| TEXAS INSTRUMENTS INCORPORATED
| Standard Linear and Logic Group
| IBIS Model of SN74CBT3125C
| QUADRUPLE FET BUS SWITCH WITH-2V UNDERSHOOT PROTECTION
| This file contains package information for the following:
|  SOIC 14-pin (D) package as [Component] CBT3125C_D
|  SSOP 14-pin (DB) package as [Component] CBT3125C_DB
|  TSSOP 14-pin (PW) package as [Component] CBT3125C_PW
|  SSOP 16-pin (DBQ) package as [Component] CBT3125C_DBQ
|  QFN 14-pin (RGY) package as [Component] CBT3125C_RGY
|  TVSOP 14-pin (DGV) package as [Component] CBT3125C_DGV
| This device can be powered at the following Vccs:
|  5 volt Vcc
|  4 volt Vcc
| This file provides unique models under the [Model Selector] for each Vcc.
| For operation at a specific Vcc, select the appropriate model after each
| [Model Selector] keyword.
[IBIS Ver]   3.2
[Comment char]  |_char
[File Name]   sn74cbt3125c.ibs
[File Rev]   1.1 | b_die
[Date]   JULY 9, 2003
[Source]   Data created from TI-SPICE simulations at TI-SLL.
[Notes]   The following is an IBIS list for the CBT3125C.
   Please contact sllibis@ti.com with questions and
   comments concerning SLL IBIS models.
   - The SSOP 16-pin package Component is commented out as
   there is different Series Pin Mapping.
   - Power-clamp data has been deleted since there is no
   power-clamp diode in the device.
   - Non-monotonic data due to FET characteristics.
[Disclaimer] Property of Texas Instruments Incorporated.  Unauthorized
   reproduction and/or distribution is strictly prohibited.
   This product is protected under copyright law.
   Created  2003, (C) Copyright  2003, Texas Instruments
   Incorporated, All Rights Reserved
   UNLESS THERE IS A SIGNED, WRITTEN AGREEMENT TO THE
   CONTRARY, TEXAS INSTRUMENTS (TI) IS PROVIDING THE IBIS
   MODELS  AND WITHOUT ANY WARRANTY, EXPRESSED OR
   IMPLIED.  TI assumes no liability for:
   1) the accuracy of the IBIS models provided to your
   company;
   2) the proper functioning of these IBIS Models in your
   design or for any resulting applications; or
   3) infringement of patents, copyrights or intellectual
   property rights resulting from your use of these IBIS
   models.
   TI provides IBIS Models as a service to our customers.
   You and your company shall not distribute, sell or give
   these models to anyone else without prior written
   permission from TI.
   TI reserves the right to make changes to our products or
   to discontinue any semiconductor product or service
   without notice, and advises our customers to obtain the
   latest version of relevant information to verify, before
   placing orders, that the information being relied on is
   current.
   Please be aware that your receipt and use of the IBIS
   information provided shall serve as acceptance of these
   terms and conditions.  If you do not accept these terms,
   you should return or destroy the IBIS models and any
   other accompanying information immediately.
| Component CBT3125C_D 14-pin SOIC
[Component]   CBT3125C_D
[Manufacturer]   Texas Instruments, Inc.
[Package]
|   typ   min   max
R_pkg   3.100e-02   2.800e-02   3.400e-02
L_pkg   3.109e-09   2.462e-09   3.889e-09
C_pkg   4.730e-13   3.630e-13   6.280e-13
[Pin]   signal_name   model_name   R_pin   L_pin   C_pin
1   1NOE   CBT3125C_IN   3.300e-02   3.854e-09   6.220e-13
2   1A   CBT3125C_IO   3.200e-02   3.188e-09   4.730e-13
3   1B   CBT3125C_IO   2.800e-02   2.462e-09   3.770e-13
4   2NOE   CBT3125C_IN   3.100e-02   2.596e-09   3.630e-13
5   2A   CBT3125C_IO   2.800e-02   2.521e-09   3.720e-13
6   2B   CBT3125C_IO   3.400e-02   3.250e-09   4.760e-13
7   GND   GND   3.400e-02   3.889e-09   6.280e-13
8   3B   CBT3125C_IO   3.400e-02   3.889e-09   6.280e-13
9   3A   CBT3125C_IO   3.400e-02   3.250e-09   4.760e-13
10   3NOE   CBT3125C_IN   2.800e-02   2.521e-09   3.720e-13
11   4B   CBT3125C_IO   3.100e-02   2.596e-09   3.640e-13
12   4A   CBT3125C_IO   2.800e-02   2.462e-09   3.770e-13
13   4NOE   CBT3125C_IN   3.200e-02   3.188e-09   4.730e-13
14   VCC   POWER   3.300e-02   3.854e-09   6.220e-13
| Component CBT3125C_DB 14-pin SSOP
[Component]   CBT3125C_DB
[Manufacturer]   Texas Instruments, Inc.
[Package]
|   typ   min   max
R_pkg   4.400e-02   4.100e-02   4.600e-02
L_pkg   3.551e-09   3.258e-09   3.927e-09
C_pkg   4.020e-13   3.600e-13   4.210e-13
[Pin]   signal_name   model_name   R_pin   L_pin   C_pin
1   1NOE   CBT3125C_IN   4.600e-02   3.927e-09   4.080e-13
2   1A   CBT3125C_IO   4.400e-02   3.587e-09   4.210e-13
3   1B   CBT3125C_IO   4.100e-02   3.289e-09   3.980e-13
4   2NOE   CBT3125C_IN   4.200e-02   3.258e-09   3.600e-13
5   2A   CBT3125C_IO   4.100e-02   3.286e-09   4.030e-13
6   2B   CBT3125C_IO   4.400e-02   3.586e-09   4.210e-13
7   GND   GND   4.600e-02   3.927e-09   4.080e-13
8   3B   CBT3125C_IO   4.600e-02   3.927e-09   4.080e-13
9   3A   CBT3125C_IO   4.400e-02   3.586e-09   4.210e-13
10   3NOE   CBT3125C_IN   4.100e-02   3.286e-09   4.030e-13
11   4B   CBT3125C_IO   4.300e-02   3.258e-09   3.600e-13
12   4A   CBT3125C_IO   4.100e-02   3.289e-09   3.980e-13
13   4NOE   CBT3125C_IN   4.400e-02   3.587e-09   4.210e-13
14   VCC   POWER   4.600e-02   3.927e-09   4.080e-13
| Component CBT3125C_DGV 14-pin TVSOP
[Component]   CBT3125C_DGV
[Manufacturer]   Texas Instruments, Inc.
[Package]
|   typ   min   max
R_pkg   3.500e-02   2.000e-02   4.500e-02
L_pkg   2.499e-09   2.077e-09   2.966e-09
C_pkg   3.610e-13   3.050e-13   4.160e-13
[Pin]   signal_name   model_name   R_pin   L_pin   C_pin
1   1NOE   CBT3125C_IN   2.700e-02   2.717e-09   3.730e-13
2   1A   CBT3125C_IO   3.700e-02   2.434e-09   3.980e-13
3   1B   CBT3125C_IO   3.400e-02   2.200e-09   3.160e-13
4   2NOE   CBT3125C_IN   2.000e-02   2.077e-09   3.090e-13
5   2A   CBT3125C_IO   3.000e-02   2.147e-09   3.050e-13
6   2B   CBT3125C_IO   4.200e-02   2.580e-09   4.080e-13
7   GND   GND   3.900e-02   2.921e-09   3.850e-13
8   3B   CBT3125C_IO   3.300e-02   2.841e-09   3.800e-13
9   3A   CBT3125C_IO   4.200e-02   2.611e-09   4.100e-13
10   3NOE   CBT3125C_IN   3.800e-02   2.331e-09   3.290e-13
11   4B   CBT3125C_IO   2.600e-02   2.223e-09   3.190e-13
12   4A   CBT3125C_IO   3.400e-02   2.259e-09   3.130e-13
13   4NOE   CBT3125C_IN   4.500e-02   2.681e-09   4.160e-13
14   VCC   POWER   4.200e-02   2.966e-09   3.860e-13
| Component CBT3125C_PW 14-pin TSSOP
[Component]   CBT3125C_PW
[Manufacturer]   Texas Instruments, Inc.
[Package]
|   typ   min   max
R_pkg   3.200e-02   2.900e-02   3.500e-02
L_pkg   2.378e-09   2.170e-09   2.680e-09
C_pkg   3.140e-13   2.700e-13   3.350e-13
[Pin]   signal_name   model_name   R_pin   L_pin   C_pin
1   1NOE   CBT3125C_IN   3.300e-02   2.618e-09   3.300e-13
2   1A   CBT3125C_IO   3.100e-02   2.313e-09   3.170e-13
3   1B   CBT3125C_IO   3.000e-02   2.310e-09   3.140e-13
4   2NOE   CBT3125C_IN   3.100e-02   2.173e-09   2.720e-13
5   2A   CBT3125C_IO   3.000e-02   2.204e-09   3.090e-13
6   2B   CBT3125C_IO   3.200e-02   2.315e-09   3.170e-13
7   GND   GND   3.500e-02   2.680e-09   3.350e-13
8   3B   CBT3125C_IO   3.300e-02   2.640e-09   3.330e-13
9   3A   CBT3125C_IO   3.400e-02   2.347e-09   3.190e-13
10   3NOE   CBT3125C_IN   2.900e-02   2.277e-09   3.130e-13
11   4B   CBT3125C_IO   3.100e-02   2.170e-09   2.700e-13
12   4A   CBT3125C_IO   3.100e-02   2.244e-09   3.110e-13
13   4NOE   CBT3125C_IN   3.300e-02   2.343e-09   3.210e-13
14   VCC   POWER   3.500e-02   2.657e-09   3.320e-13
| NOTE: 16-pin SSOP Component package is commented out below because different
| Series pin mapping for the 16 vs 14 pin package
| Component CBT3125C_RGY 14-pin QFN
[Component]   CBT3125C_RGY
[Manufacturer]   Texas Instruments, Inc.
[Package]
|   typ   min   max
R_pkg   2.900e-02   2.300e-02   4.100e-02
L_pkg   7.730e-10   6.570e-10   9.980e-10
C_pkg   1.360e-13   1.150e-13   1.560e-13
[Pin]   signal_name   model_name   R_pin   L_pin   C_pin
1   1NOE   CBT3125C_IN   2.700e-02   8.310e-10   1.300e-13
2   1A   CBT3125C_IO   2.700e-02   8.660e-10   1.350e-13
3   1B   CBT3125C_IO   4.100e-02   9.980e-10   1.560e-13
4   2NOE   CBT3125C_IN   3.100e-02   7.670e-10   1.420e-13
5   2A   CBT3125C_IO   3.100e-02   7.650e-10   1.420e-13
6   2B   CBT3125C_IO   3.100e-02   7.830e-10   1.440e-13
7   GND   GND   3.100e-02   7.810e-10   1.370e-13
8   3B   CBT3125C_IO   2.300e-02   6.570e-10   1.150e-13
9   3A   CBT3125C_IO   2.300e-02   8.140e-10   1.290e-13
10   3NOE   CBT3125C_IN   2.800e-02   7.040e-10   1.290e-13
11   4B   CBT3125C_IO   2.700e-02   6.720e-10   1.360e-13
12   4A   CBT3125C_IO   2.700e-02   6.960e-10   1.380e-13
13   4NOE   CBT3125C_IN   2.700e-02   7.250e-10   1.400e-13
14   VCC   POWER   3.000e-02   7.630e-10   1.360e-13
|| Component CBT3125C_DBQ 16-pin SSOP
|[Component]   CBT3125C_DBQ
|[Manufacturer]   Texas Instruments, Inc.
|[Package]
||   typ   min   max
|R_pkg   3.800e-02   2.700e-02   5.900e-02
|L_pkg   2.353e-09   1.491e-09   4.500e-09
|C_pkg   2.100e-13   6.400e-14   5.920e-13
|[Pin]   signal_name   model_name   R_pin   L_pin   C_pin
|1   NC   NC   5.800e-02   4.450e-09   5.920e-13
|2   1NOE   CBT3125C_IO   4.000e-02   1.930e-09   1.110e-13
|3   1A   CBT3125C_IO   2.800e-02   1.538e-09   7.600e-14
|4   1B   CBT3125C_IO   2.700e-02   1.491e-09   6.400e-14
|5   2NOE   CBT3125C_IO   2.700e-02   1.491e-09   6.400e-14
|6   2A   CBT3125C_IO   2.700e-02   1.506e-09   7.500e-14
|7   2B   CBT3125C_IO   3.300e-02   1.922e-09   1.090e-13
|8   GND   GND   5.900e-02   4.500e-09   5.880e-13
|9   NC   NC   5.800e-02   3.695e-09   4.140e-13
|10   3B   CBT3125C_IO   3.400e-02   2.685e-09   2.820e-13
|11   3A   CBT3125C_IO   2.900e-02   1.552e-09   7.700e-14
|12   3NOE   CBT3125C_IO   2.800e-02   1.506e-09   6.500e-14
|13   4B   CBT3125C_IO   2.700e-02   1.492e-09   6.400e-14
|14   4A   CBT3125C_IO   2.800e-02   1.534e-09   7.600e-14
|15   4NOE   CBT3125C_IO   4.000e-02   2.703e-09   2.840e-13
|16   VCC   POWER   5.600e-02   3.645e-09   4.180e-13
[Series Switch Groups]
| Function Group States
On  1 /   | 1a->1b 1noe low
On  2 /   | 2a->2b 2noe low
On  3 /   | 3a->3b 3noe low
On  4 /   | 4a->4b 4noe low
On  1 2 /   | 1noe low, 2noe low
On  1 3 /   | 1noe low, 3noe low
On  1 4 /   | 1noe low, 4noe low
On  2 3 /   | 2noe low, 3noe low
On  2 4 /   | 2noe low, 4noe low
On  3 4 /   | 4noe low, 3noe low
On  1 2 3 /   | 1noe low, 2noe low, 3noe low
On  1 2 4 /   | 1noe low, 2noe low, 4noe low
On  1 3 4 /   | 1noe low, 3noe low, 4noe low
On  1 2 3 4  /   | 1noe low, 2noe low, 3noe low, 4noe low Enable all
Off 1 2 3 4 /   | 1noe high, 2noe high, 3noe high, 4noe high Disable all
[Series Pin Mapping]   pin_2   model_name   function_table_group
2   3   CBT3125C_IO_50_S   1
| 2   3   CBT3125C_IO_40_S   1
5   6   CBT3125C_IO_50_S   2
| 5   6   CBT3125C_IO_40_S   2
9   8   CBT3125C_IO_50_S   3
| 9   8   CBT3125C_IO_40_S   3
12   11   CBT3125C_IO_50_S   4
| 12   11   CBT3125C_IO_40_S   4
|  NOTE, this series mapping is for the SSOP 16 pin Component
|3   4   CBT3125C_IO_50_S   1
|| 3   4   CBT3125C_IO_40_S   1
|6   7   CBT3125C_IO_50_S   2
|| 6   7   CBT3125C_IO_40_S   2
|11   10   CBT3125C_IO_50_S   3
|| 11   10   CBT3125C_IO_40_S   3
|14   13   CBT3125C_IO_50_S   4
|| 14   13   CBT3125C_IO_40_S   4
| Model CBT3125C_IN
[Model Selector]   CBT3125C_IN
CBT3125C_IN_50   5 volt Vcc
CBT3125C_IN_40   4 volt Vcc
| Model CBT3125C_IO
[Model Selector]   CBT3125C_IO
CBT3125C_IO_50   5 volt Vcc
CBT3125C_IO_40   4 volt Vcc
| Model CBT3125C_IO_S
[Model Selector]   CBT3125C_IO_S
CBT3125C_IO_50_S   5 volt Vcc_S
CBT3125C_IO_40_S   4 volt Vcc_S
[Model]   CBT3125C_IO_50_S
Model_type  Series_switch
| variable   typ   min   max
C_comp   0   0   0
[Temperature Range]   40   100   -40
| Ambient temperature   25   85   -40
[Voltage range]   5   4.5   5.5
[On]
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[Off]
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[Model]   CBT3125C_IO_40_S
Model_type  Series_switch
| variable   typ   min   max
C_comp   0   0   0
[Temperature Range]   40   100   -40
| Ambient temperature   25   85   -40
[Voltage range]   4   4   4
[On]
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[Off]
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| Models and submodels in the file (6): CBT3125C_IN_50 (Input), CBT3125C_IN_40 (Input), CBT3125C_IO_50_S (Series_switch), CBT3125C_IO_50 (Terminator), CBT3125C_IO_40_S (Series_switch), CBT3125C_IO_40 (Terminator)
